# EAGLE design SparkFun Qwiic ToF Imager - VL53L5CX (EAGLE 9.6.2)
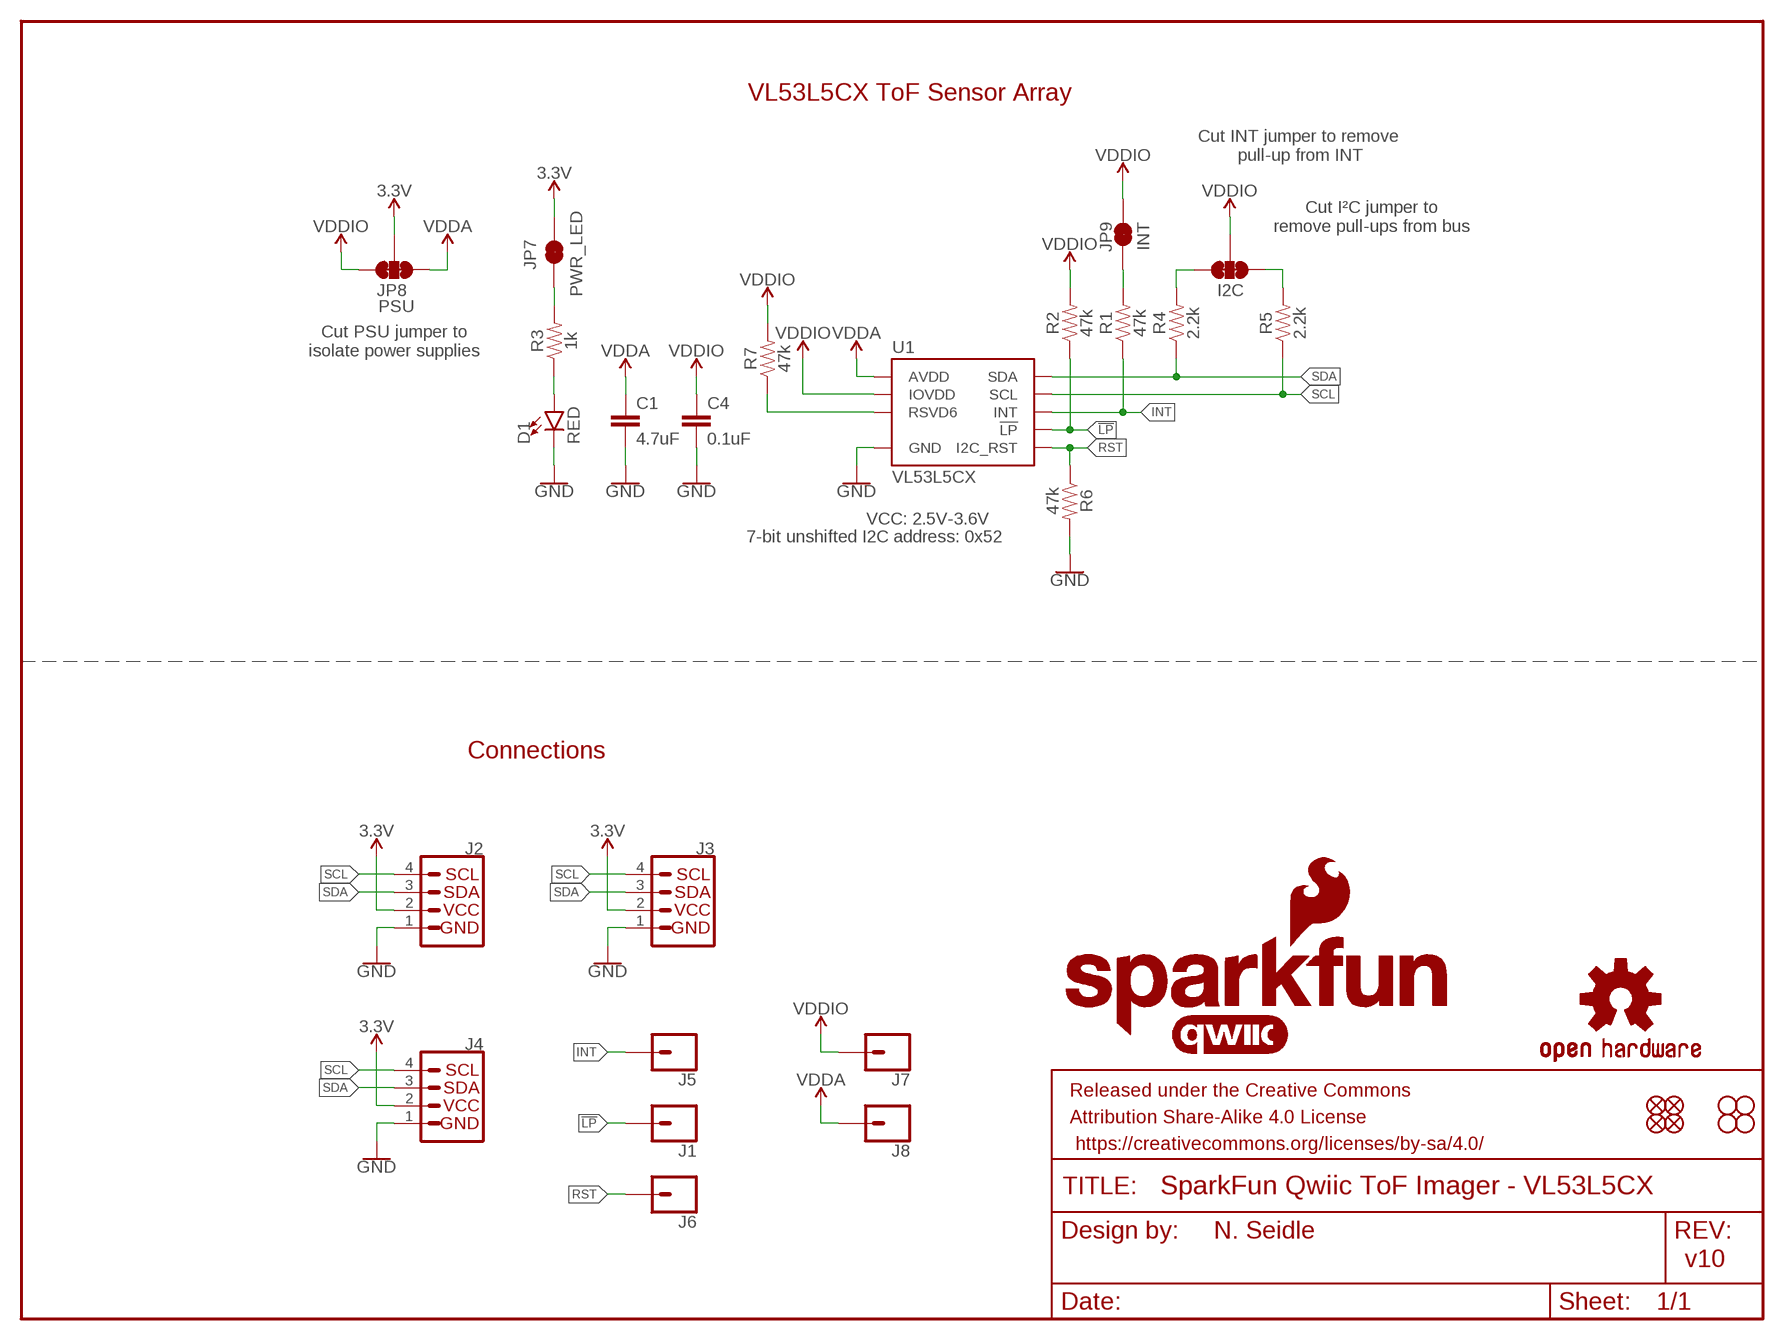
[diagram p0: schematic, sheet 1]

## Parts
C1  4.7uF  4.7UF-0603-6.3V-(10%)  [0603]
C4  0.1uF  0.1UF-0603-25V-(+80/-20%)  [0603]
D1  RED  LED-RED0603  [LED-0603]
FRAME1  FRAME-LETTER  [CREATIVE_COMMONS]
I2C  JUMPER-SMT_3_2-NC_TRACE_SILK  [SMT-JUMPER_3_2-NC_TRACE_SILK]
J1  CONN_01PTH_NO_SILK_YES_STOP  [1X01_NO_SILK]
J2  QWIIC_CONNECTORJS-1MM  [JST04_1MM_RA]
J3  PTH  I2C_STANDARD_NO_SILK  [1X04_NO_SILK]
J4  QWIIC_CONNECTORJS-1MM  [JST04_1MM_RA]
J5  CONN_01PTH_NO_SILK_YES_STOP  [1X01_NO_SILK]
J6  CONN_01PTH_NO_SILK_YES_STOP  [1X01_NO_SILK]
J7  CONN_01PTH_NO_SILK_YES_STOP  [1X01_NO_SILK]
J8  CONN_01PTH_NO_SILK_YES_STOP  [1X01_NO_SILK]
JP1  FIDUCIALUFIDUCIAL  [MICRO-FIDUCIAL]
JP2  FIDUCIALUFIDUCIAL  [MICRO-FIDUCIAL]
JP3  STAND-OFF  [STAND-OFF]
JP4  STAND-OFF  [STAND-OFF]
JP5  FIDUCIALUFIDUCIAL  [MICRO-FIDUCIAL]
JP6  FIDUCIALUFIDUCIAL  [MICRO-FIDUCIAL]
JP7  PWR_LED  JUMPER-SMT_2_NC_TRACE_SILK  [SMT-JUMPER_2_NC_TRACE_SILK]
JP8  PSU  JUMPER-SMT_3_2-NC_TRACE_SILK  [SMT-JUMPER_3_2-NC_TRACE_SILK]
JP9  INT  JUMPER-SMT_2_NC_TRACE_SILK  [SMT-JUMPER_2_NC_TRACE_SILK]
JP10  STAND-OFF  [STAND-OFF]
JP11  STAND-OFF  [STAND-OFF]
LOGO1  OSHW-LOGOMINI  [OSHW-LOGO-MINI]
LOGO3  QWIIC_LOGO_CONNECTOR  [QWIIC_5.5MM]
R1  47k  47KOHM-0603-1/10W-1%  [0603]
R2  47k  47KOHM-0603-1/10W-1%  [0603]
R3  1k  1KOHM-0603-1/10W-1%  [0603]
R4  2.2k  2.2KOHM-0603-1/10W-1%  [0603]
R5  2.2k  2.2KOHM-0603-1/10W-1%  [0603]
R6  47k  47KOHM-0603-1/10W-1%  [0603]
R7  47k  47KOHM-0603-1/10W-1%  [0603]
U1  VL53L5CX  [VL53L5CX]
U$1  SFE_LOGO_NAME.1_INCH  [SFE_LOGO_NAME_.1]
U$2  SFE_LOGO_NAME_FLAME.1_INCH  [SFE_LOGO_NAME_FLAME_.1]

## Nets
3.3V: J2.2 J3.2(VCC) J4.2 JP7.2 JP8.2
!LP: J1.1 R2.1 U1.A5(!LP)
GND: C1.2 C4.2 D1.C J2.1 J3.1(GND) J4.1 R6.2 U1.A2(GND) U1.A6(GND) U1.A7(GND) U1.B4(GND) U1.C1(GND) U1.C6(GND) U1.C7(GND)
INT: J5.1 R1.1 U1.A3(INT)
N$1: I2C.1 R5.2
N$2: I2C.3 R4.2
N$3: D1.A R3.1
N$4: JP9.1 R1.2
N$5: JP7.1 R3.2
N$6: R7.1 U1.C2(RSVD6)
RST: J6.1 R6.1 U1.A1(I2C_RST)
SCL: J2.4 J3.4(SCL) J4.4 R5.1 U1.C4(SCL)
SDA: J2.3 J3.3(SDA) J4.3 R4.1 U1.C3(SDA)
VDDA: C1.1 J8.1 JP8.1 U1.B1(AVDD) U1.B7(AVDD)
VDDIO: C4.1 I2C.2 J7.1 JP8.3 JP9.2 R2.2 R7.2 U1.A4(IOVDD)

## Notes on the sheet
- VL53L5CX ToF Sensor Array
- Cut INT jumper to remove 
  pull-up from INT
- Cut I²C jumper to
  remove pull-ups from bus
- Cut PSU jumper to
  isolate power supplies
- VCC: 2.5V-3.6V
- 7-bit unshifted I2C address: 0x52
- Connections
- N. Seidle
- v10

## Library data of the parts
C1 = SparkFun-Capacitors:4.7UF: 4.7µF ceramic capacitors; PROD_ID: CAP-08280
C4 = SparkFun-Capacitors:0.1UF: 0.1µF ceramic capacitors; PROD_ID: CAP-00810
D1 = SparkFun-LED:LED-RED: Red SMD LED; PROD_ID: DIO-00819
FRAME1 = SparkFun-Aesthetics:FRAME-LETTER: Schematic Frame - Letter
I2C JP8 = SparkFun-Jumpers:JUMPER-SMT_3_2-NC_TRACE: Normally closed trace jumper (2 of 2 connections) This jumper has a trace between all three pads so they are normally closed (NC). Use a razor knife to open the connection(s). For best results follow the IPC guidelines for cutting traces: Cutout at least 0.063 mm (0.005 in). Remove all loose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
J1 J5-J8 = SparkFun-Connectors:CONN_01: Single connection point. Often used as Generic Header-pin footprint for 0.1 inch spaced/style header connections
J2 J4 = SparkFun-Connectors:QWIIC_CONNECTOR: SparkFun I2C Standard Qwiic Connector An SMD 1mm pitch JST connector makes it easy and quick (get it? Qwiic?) to connect I2C devices to each other. The Qwiic system enables fast and solderless connection between popular platforms and various sensors and actuators. We carry 200mm, 100mm, 50mm, and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; PROD_ID: CONN-13694; VALUE: QWIIC_RIGHT_ANGLE
J3 = SparkX:I2C_STANDARD: SparkFun I2C Standard Pinout Header SparkFun has standardized on a pinout for all I2C based sensor breakouts. This pinout allows I2C boards to be plugged directly into the headers on Arduino Uno compatible boards, and to be daisy chained easily. Example SparkFun Products: SparkFun Atmospheric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
JP1 JP2 JP5 JP6 = SparkFun:FIDUCIAL: Fiducial Alignment Points
JP3 JP4 JP10 JP11 = SparkFun:STAND-OFF: Stand Off
JP7 JP9 = SparkFun-Jumpers:JUMPER-SMT_2_NC_TRACE: Normally closed trace jumper
LOGO1 = SparkFun-Aesthetics:OSHW-LOGO: Open-Source Hardware (OSHW) Logo
LOGO3 = SparkFun-Aesthetics:QWIIC_LOGO: Qwiic Logos for placement on schematic and PCB. The 5.5mm silk logo is best for placing next to Qwiic connector.
R1 R2 R6 R7 = SparkFun-Resistors:47KOHM: 47kΩ resistor; PROD_ID: RES-07871
R3 = SparkFun-Resistors:1KOHM: 1kΩ resistor; PROD_ID: RES-07856
R4 R5 = SparkFun-Resistors:2.2KOHM: 2.2kΩ resistor; PROD_ID: RES-08272
U1 = SparkFun-Sensors:VL53L5CX; PROD_ID: IC-16254
U$1 = SparkFun-Aesthetics:SFE_LOGO_NAME: SparkFun Font Logo
U$2 = SparkFun-Aesthetics:SFE_LOGO_NAME_FLAME: SparkFun Font Logo w/ Flame

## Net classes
1 power: width 0.203 mm

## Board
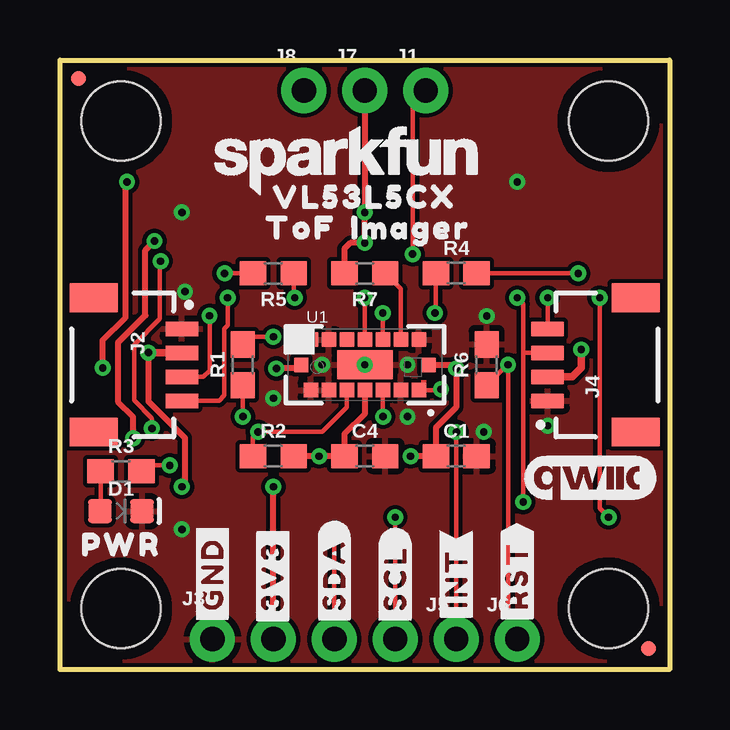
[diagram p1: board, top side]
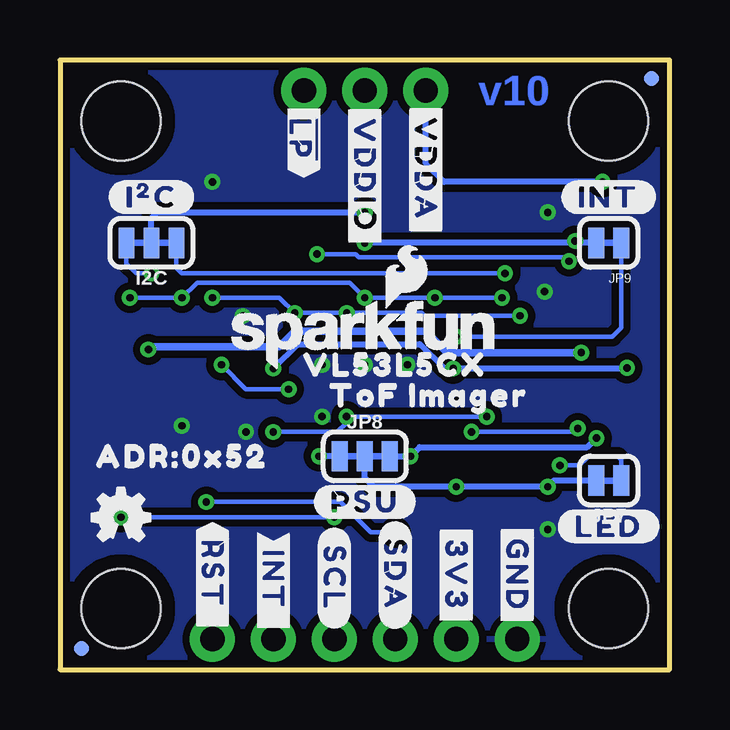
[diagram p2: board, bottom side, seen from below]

Size 25.4 x 25.4 mm. Coordinates in mm from the lower left corner, seen from the top.
Outline: 0,0 0,25.4 25.4,25.4 25.4,0 0,0
Copper layers (1*16): Top/Vert 0.035mm / dielectric 1.5mm / Bottom/Horz 0.035mm
Design rules "SparkFun-2-Layer-General-JLCPCB": minimum track width 7mil, minimum drill 0.3mm, track to track 7mil, track to pad 7mil, pad to pad 7mil, via to via 7mil, smd to smd 7mil, copper to edge 7mil, drill to drill 7mil, minimum pad ring 7mil, minimum via ring 7mil, stop-mask expansion 3mil, vias tented up to drill 25mil, thermal gap 10mil

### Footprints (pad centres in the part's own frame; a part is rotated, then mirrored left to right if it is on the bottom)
0603 = smd 1.1 x 1: 1 -0.85,0; 2 0.85,0
LED-0603 = smd 1 x 1: A -0.877,0; C 0.877,0
SMT-JUMPER_3_2-NC_TRACE_SILK = smd 0.66 x 1.27: 1 -1.041,0; 2 0,0; 3 1.041,0
1X01_NO_SILK = drill 1.016 pad 1.88: 1 0,0
JST04_1MM_RA = smd 0.6 x 1.35: 1 -1.5,0; 2 -0.5,0; 3 0.5,0; 4 1.5,0 | smd 1.2 x 2: NC1 2.8,-3.675; NC2 -2.8,-3.675
1X04_NO_SILK = drill 1.016 pad 1.88: 1 0,0; 2 2.54,0; 3 5.08,0; 4 7.62,0
MICRO-FIDUCIAL = smd 0.635 x 0.635: 1 0,0
STAND-OFF = hole 3.302: 0,0
SMT-JUMPER_2_NC_TRACE_SILK = smd 0.66 x 1.27: 1 -0.521,0; 2 0.521,0
VL53L5CX = smd 0.6 x 0.6: A1 2.25,-1.05; A2 1.5,-1.05; A3 0.75,-1.05; A4 0,-1.05; A5 -0.75,-1.05; A6 -1.5,-1.05; A7 -2.25,-1.05; B1 2.65,0; B7 -2.65,0; C1 2.25,1.05; C2 1.5,1.05; C3 0.75,1.05; C4 0,1.05; C5 -0.75,1.05; C6 -1.5,1.05; C7 -2.25,1.05 | smd 2.316 x 1.2: B4 0,0

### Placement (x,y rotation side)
C1  16.51,8.89 0 top
C4  12.7,8.89 0 top
D1  2.54,6.6 0 top
FRAME1  not placed on the board
I2C  21.59,17.78 180 bottom
J1  15.24,24.13 0 top
J2  5.08,12.7 270 top
J3  6.35,1.27 0 top
J4  20.32,12.7 90 top
J5  16.51,1.27 0 top
J6  19.05,1.27 0 top
J7  12.7,24.13 0 top
J8  10.16,24.13 0 top
JP1  0.76,24.64 0 bottom
JP2  24.51,0.89 0 top
JP3  2.54,22.86 0 top
JP4  22.86,22.86 0 top
JP5  24.51,0.89 0 bottom
JP6  0.76,24.64 0 top
JP7  2.54,7.87 180 bottom
JP8  12.7,8.89 0 bottom
JP9  2.54,17.78 180 bottom
JP10  2.54,2.54 0 top
JP11  22.86,2.54 0 top
LOGO1  22.86,6.35 0 bottom
LOGO3  22.1,8 0 top
R1  7.62,12.7 90 top
R2  8.89,8.89 0 top
R3  2.54,8.26 0 top
R4  16.51,16.51 0 top
R5  8.89,16.51 180 top
R6  17.78,12.7 90 top
R7  12.7,16.51 180 top
U1  12.7,12.7 0 top
U$1  11.94,21.21 0 top
U$2  12.7,13.97 0 bottom
U$3  [#3V3#13]  8.89,3.94 270 bottom
U$4  [PWR12]  2.54,5.21 0 top
U$5  [#LED#10]  2.54,5.97 0 bottom
U$6  [#INT#0]  16.51,3.81 90 top
U$7  [#RST#1]  19.05,3.94 90 top
U$8  [#INT_#0]  16.51,3.56 270 bottom
U$9  [#RST_#1]  19.05,3.81 270 bottom
U$10  [##LP##2]  15.24,22.1 270 bottom
U$11  [#INT#1]  2.54,19.68 0 bottom
U$12  [#VDDA#0]  10.16,20.83 270 bottom
U$13  [ADR#0X520]  20.32,8.89 0 bottom
U$14  [#VDDIO#1]  12.7,20.57 270 bottom
U$15  [#PSU#0]  12.7,6.99 0 bottom
U$16  [#I�C#0]  21.59,19.68 0 bottom
U$17  [VL53L5CX0]  12.7,19.68 0 top
U$18  [IMAGER2]  14.61,18.41 0 top
U$19  [VL53L5CX0]  11.43,12.7 0 bottom
U$20  [TOF1]  12.7,11.43 0 bottom
U$21  [#3V3#13]  8.86,3.89 90 top
U$22  [IMAGER2]  8.38,11.43 0 bottom
U$23  [TOF1]  10.03,18.41 0 top
U$24  [#SCL#1]  13.97,3.81 270 bottom
U$25  [#SDA#0]  11.43,3.94 270 bottom
U$26  [#GND#62130]  6.35,3.99 90 top
U$28  [#SDA#62131]  11.43,3.96 90 top
U$29  [#SCL#62132]  13.97,3.81 90 top
U$30  [#GND#62130]  6.35,3.94 270 bottom

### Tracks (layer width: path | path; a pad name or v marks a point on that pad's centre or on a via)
3.3V  (via drill 0.3)
  Top/Vert 0.254: J3.2 v8.89,7.62 | v3.68,13.21 3.68,11.18 5.21,9.65 5.21,7.75 v5.08,7.62
  Top/Vert 0.305: J2.2 3.69,13.2 v3.68,13.21 | v21.72,13.34 21.72,12.57 21.34,12.2 J4.2
  Bottom/Horz 0.254: JP7.2 4.83,7.87 v5.08,7.62 v8.89,7.62 12.32,7.62 12.7,8 JP8.2
  Bottom/Horz 0.305: v3.68,13.21 9.27,13.21 10.16,14.1 15.62,14.1 16.26,13.46 21.59,13.46 v21.72,13.34
!LP  (via drill 0.3)
  Top/Vert 0.178: U1.A5 11.95,10.93 10.92,9.91 v8.26,9.91 8.04,9.69 R2.1 | J1.1 14.69,23.58 v14.69,17.31 | v3.83,10.05 3.83,10.47 3.09,11.22 3.09,13.54 4.15,14.61 4.15,16.98 v4.19,17.02
  Bottom/Horz 0.178: v14.69,17.31 13.07,17.31 12.95,17.18 4.36,17.18 v4.19,17.02 | v8.26,9.91 3.97,9.91 v3.83,10.05
GND  (via drill 0.3)
  other vias: 20.32,10.16 17.78,14.73 14.48,10.54 17.65,9.91 5.08,5.84 10.92,12.7 14.48,12.7 12.7,12.7 5.21,15.75 8.89,11.3 5.08,19.05 19.05,20.32
  pour Bottom/Horz (isolate 0.305): 0,0 0,25.4 25.4,25.4 25.4,0
  pour Top/Vert (isolate 0.178): 0,0 0,25.4 25.4,25.4 25.4,0
INT  (via drill 0.3)
  Top/Vert 0.178: U1.A3 13.45,10.55 v13.46,10.54 | v7.62,10.54 R1.1 | J5.1 v16.51,9.9 v16.52,9.9
  Bottom/Horz 0.178: v7.62,10.54 v13.46,10.54 13.46,10.29 13.85,9.9 v16.52,9.9
N$1  (via drill 0.3)
  Top/Vert 0.178: R5.2 v6.86,16.51
  Bottom/Horz 0.178: v6.86,16.51 20.32,16.51 20.55,16.74 I2C.1
N$2  (via drill 0.3)
  Top/Vert 0.178: R4.2 v21.59,16.51
  Bottom/Horz 0.178: v21.59,16.51 22.23,16.51 22.63,16.92 I2C.3
N$3
  Top/Vert 0.178: R3.1 1.69,6.63 D1.A
N$4  (via drill 0.3)
  Top/Vert 0.178: R1.2 7.94,13.87 v8.89,13.87
  Bottom/Horz 0.178: v8.89,13.87 2.54,13.87 2.44,13.87 2.39,13.87 2.02,14.24 JP9.1
N$5  (via drill 0.3)
  Top/Vert 0.178: R3.2 3.64,8.51 v4.57,8.51
  Bottom/Horz 0.178: v4.57,8.51 3.77,8.51 3.4,8.88 2.15,8.88 2.02,8.75 JP7.1
N$6
  Top/Vert 0.178: U1.C2 14.2,15.86 R7.1
RST  (via drill 0.3)
  Top/Vert 0.178: U1.A1 15.88,11.65 v15.88,11.68 | R6.1 18.63,12.7 v18.67,12.7 18.67,1.65 J6.1
  Bottom/Horz 0.178: v18.67,12.7 17.65,11.68 v15.88,11.68
SCL  (via drill 0.3)
  Top/Vert 0.178: U1.C4 v12.7,15.49 | v20.32,15.49 J4.4 | R5.1 9.74,15.53 v9.78,15.49 | v6.99,15.49 6.99,14.34 6.85,14.21 6.85,11.43 6.63,11.2 J2.4 | J3.4 v13.97,6.35 | v22.86,6.35 22.49,6.72 v22.49,15.49
  Bottom/Horz 0.178: v6.99,15.49 v9.78,15.49 v12.7,15.49 13.34,16.13 19.68,16.13 v20.32,15.49 v22.49,15.49 | v13.97,6.35 v22.86,6.35
SDA  (via drill 0.3)
  Top/Vert 0.178: U1.C3 v13.45,14.86 | R4.1 15.66,14.9 v15.62,14.86 | J2.3 5.98,12.2 6.23,12.46 v6.23,14.74 | J3.3 v11.43,5.71 | v19.05,15.49 19.3,15.24 19.3,13.21 | v19.3,6.99 19.3,13.21 | J4.3 19.31,13.2 19.3,13.21
  Bottom/Horz 0.178: v19.05,15.49 16.26,15.49 v15.62,14.86 v13.45,14.86 10.33,14.86 10.21,14.74 v6.23,14.74 | v11.43,5.71 12.45,5.71 13.72,6.99 v19.3,6.99
VDDA  (via drill 0.3)
  Top/Vert 0.254: U1.B1 16.38,12.7 16.51,12.57 v16.51,12.55 16.51,10.92 15.66,10.07 C1.1 v14.61,8.89 | U1.B7 9.9,12.55 v9.02,12.55 | v1.78,12.57 1.78,13.71 2.71,14.65 2.71,20.24 v2.79,20.32
  Bottom/Horz 0.254: JP8.1 v14.61,8.89 | v16.51,12.55 15.49,13.56 10.41,13.56 9.4,12.55 v9.02,12.55 1.8,12.55 v1.78,12.57 | v2.79,20.32 9.4,20.32 10.16,21.08 J8.1
VDDIO  (via drill 0.3)
  Top/Vert 0.254: J7.1 v12.7,19.05 v12.7,17.78 12.1,17.78 11.85,17.53 R7.2 | U1.A4 12.7,10.67 11.85,9.82 C4.1 v10.79,8.89 R2.2 | v3.05,9.64 3.05,10.53 2.41,11.17 2.41,13.61 3.56,14.76 3.56,17.48 v3.94,17.86
  Bottom/Horz 0.254: JP8.3 v10.79,8.89 10.41,9.27 3.42,9.27 v3.05,9.64 | I2C.2 21.59,18.8 21.34,19.05 v12.7,19.05 | JP9.2 3.94,17.78 | 3.94,17.78 v12.7,17.78 | v3.94,17.86 3.94,17.78

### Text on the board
Bottom/Horz: v10
tDocu: N. Seidle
